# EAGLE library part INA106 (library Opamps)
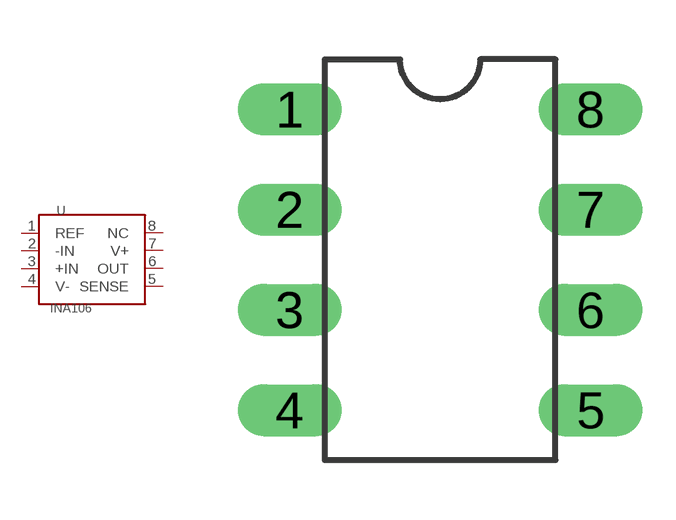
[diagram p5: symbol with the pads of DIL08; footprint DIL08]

Designator prefix U

## INA106  [DIL08]
1  REF
2  -IN
3  +IN
4  V-
5  SENSE
6  OUT
7  V+
8  NC

## Footprint DIL08 (pad centres in mm)
drill 0.813 long: 1 -3.81,3.81; 2 -3.81,1.27; 3 -3.81,-1.27; 4 -3.81,-3.81; 5 3.81,-3.81; 6 3.81,-1.27; 7 3.81,1.27; 8 3.81,3.81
